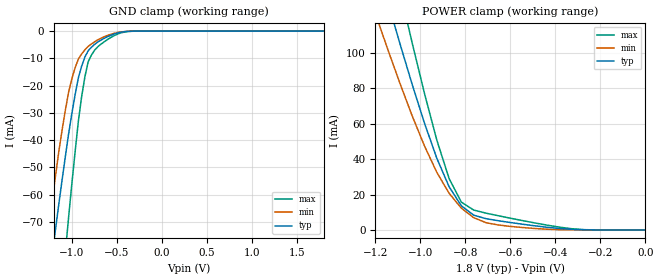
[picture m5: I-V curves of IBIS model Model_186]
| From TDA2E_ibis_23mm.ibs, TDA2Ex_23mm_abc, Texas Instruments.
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| Model based on original model for IQ1833DVTCKPBFBP18LL_SSCEV
|   Sub model IQ1833_V_10P_1P8
[model]   Model_186
|[Description]  [1.8V-INPUT-X-1.8V MODE, IND, 10 PERCENT%]
|   1.8V MODE, ,IND,10 PERCENT%
|[Input Load]
|[Output Drive] 1.8V MODE
|Voltage   1.8V
|Mode   INPUT
Model_type   Input
Polarity   Non-Inverting
Vinl =  0.306
Vinh =  1.206
C_comp   628.403f   564.553f   692.253f
[Model Spec]
Vinl   0.306   0.2754   0.3366
Vinh   1.206   1.0854   1.3266
D_overshoot_ampl_h 0.36 0.36 0.36
D_overshoot_ampl_l 0.36 0.36 0.36
D_overshoot_area_h 0.33n 0.33n 0.33n
D_overshoot_area_l 0.33n 0.33n 0.33n
D_overshoot_high 2.16 2.16 2.16
D_overshoot_low -0.36 -0.36 -0.36
D_overshoot_time 1n 1n 1n
S_overshoot_high 1.8 1.8 1.8
S_overshoot_low 0 0 0
[Temperature Range]   25   125   -40
[Voltage Range]   1.8   1.62   1.98
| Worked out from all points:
|   GND clamp passes 1 mA (typ) near -0.52 V on its own axis
|   POWER clamp passes 1 mA (typ) near -0.39 V on its own axis
[POWER_clamp]
-1.8V     435.3mA    358.7mA    550.4mA
-1.182V   145.1mA    115.2mA    186mA
-1.164V   136.9mA    108.6mA    175.7mA
-1.109V   112.9mA    89.04mA    145.1mA
-1.055V   89.59mA    70.35mA    115.1mA
-927.3mV  40.44mA    32.49mA    50.68mA
-872.7mV  24.38mA    20.69mA    29mA
-818.2mV  13.61mA    12.29mA    15.69mA
-763.6mV  8.369mA    6.955mA    11.25mA
-654.5mV  5.219mA    2.81mA     8.042mA
-327.3mV  349.6uA    49.2uA     692.7uA
0V        2.268uA    679.7nA    6.102uA
[GND_clamp]
-1.8V     -241.7mA   -231.6mA   -367.4mA
-1.255V   -91.62mA   -71.7mA    -149.9mA
-1.182V   -72.85mA   -53.19mA   -122mA
-1.073V   -46.19mA   -29.16mA   -81.51mA
-1.036V   -37.83mA   -22.49mA   -68.45mA
-927.3mV  -17.13mA   -10.25mA   -33.06mA
-890.9mV  -12.84mA   -8.372mA   -24.01mA
-818.2mV  -7.187mA   -5.618mA   -11.22mA
-745.5mV  -4.828mA   -3.892mA   -6.943mA
-563.6mV  -1.493mA   -1.146mA   -2.288mA
-381.8mV  -98.54uA   -88.38uA   -167.6uA
1.8V      2.268uA    1.69uA     5.679uA
